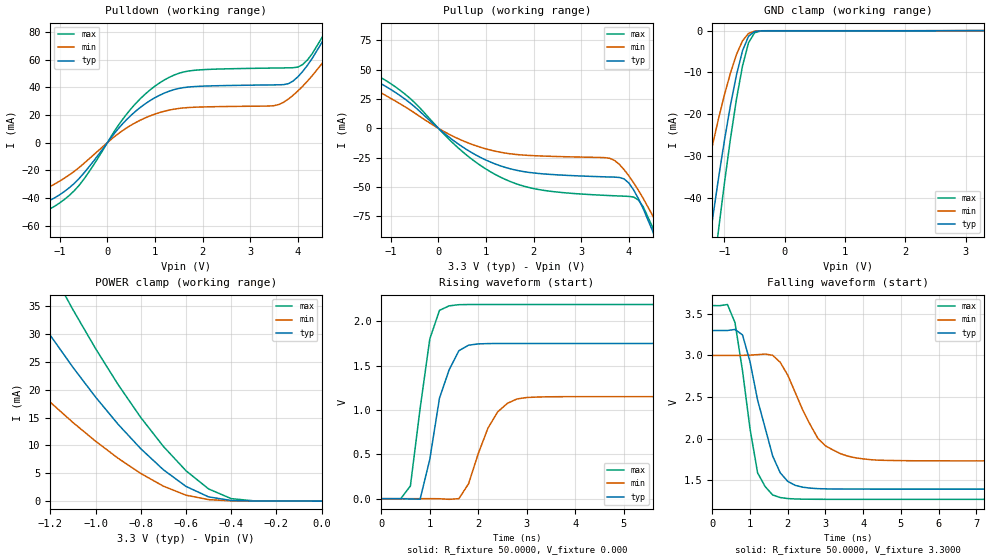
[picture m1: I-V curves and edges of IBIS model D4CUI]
| IBIS file t4i.ibs created by s2ibis2 version 1.1
| North Carolina State University Electronics Research Laboratory  1995
[IBIS ver]   2.1
[File name]   d4cui.ibs
[File Rev]   1.0
[Date]   Wednesday, March 29, 2000
[Source]   From silicon level SPICE at TOSHIBA.
[Notes]   This model does not include the values of Package Model
[Disclaimer]   None.
[Copyright]   Copyright(C) TOSHIBA Corp. 1996-2000. All Rights Reserved
|   Component TC260C
[Component]   TC260C
[Manufacturer]   TOSHIBA
[Package]
| variable   typ   min   max
R_pkg   1.00f   NA   NA
L_pkg   1.00fH   NA   NA
C_pkg   1.00fF   NA   NA
[Pin]  signal_name   model_name   R_pin   L_pin   C_pin
IO   IO   D4CUI
VDDS   VDDS   POWER
VSS   VSS   GND
| Models and submodels in the file (1): D4CUI (I/O)
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|   Model D4CUI
[Model]   D4CUI
Model_type   I/O
Polarity   Non-Inverting
Vinl   = 0.66V
Vinh   = 2.64V
C_comp   4.3pF   NA   NA
Vmeas = 1.65V
|Variable   typ   min   max
[Voltage range]  3.3   3.0   3.6
[Temperature Range]   25   100   0
[Pullup Reference]   3.3   3.0   3.6
[Pulldown Reference]   0.0   0.0   0.0
[POWER Clamp Reference]   3.3   3.0   3.6
[GND Clamp Reference]   0.0   0.0   0.0
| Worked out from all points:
|   slope of the pulldown table from 0 to 0.495 V, typ, clamps not added: 25.2 ohm
|   slope of the pullup table from 0 to 0.495 V, typ, clamps not added: 31.9 ohm
|   GND clamp passes 1 mA (typ) near -0.57 V on its own axis
|   POWER clamp passes 1 mA (typ) near -0.51 V on its own axis
|   rising waveform, R_fixture 50.0000, V_fixture 0.000: 20-80 % time 408ps typ, 500ps min, 320ps max; typ from 0 V to 1.75 V
|   falling waveform, R_fixture 50.0000, V_fixture 3.3000: 20-80 % time 615ps typ, 821ps min, 454ps max; typ from 3.3 V to 1.39 V
[Pulldown]
| voltage   I(typ)   I(min)   I(max)
-3.3V     -59mA      -58.31mA   -64.86mA
-1.9V     -51.23mA   -43.07mA   -57.58mA
-1V       -37.65mA   -27.81mA   -43.59mA
-500mV    -22.31mA   -15.25mA   -26.74mA
600mV     22.86mA    14.58mA    28.46mA
1.4V      38.26mA    24.15mA    48.77mA
3.6V      41.74mA    27.49mA    53.92mA
3.8V      42.56mA    31.44mA    54.02mA
4.1V      51.34mA    40.69mA    56.35mA
4.7V      84.91mA    66.18mA    89.44mA
5.1V      114.3mA    87.51mA    123mA
6.6V      274.3mA    211.8mA    309.5mA
[Pullup]
| voltage   I(typ)   I(min)   I(max)
-3.3V     71.91mA    86.68mA    73.87mA
-2.1V     55.22mA    51.34mA    59.93mA
-1.1V     35.6mA     27.85mA    40.67mA
-500mV    18.41mA    13.14mA    21.98mA
500mV     -15.68mA   -10.38mA   -19.73mA
1.5V      -34.43mA   -21.67mA   -45.26mA
3.7V      -41.64mA   -27.45mA   -57.55mA
4V        -46.74mA   -40.6mA    -58.07mA
4.2V      -60.02mA   -52.9mA    -61.17mA
4.5V      -87.85mA   -74.56mA   -84.58mA
4.7V      -109.3mA   -90.59mA   -107mA
6.6V      -337.2mA   -276.9mA   -360.7mA
[GND_clamp]
| voltage   I(typ)   I(min)   I(max)
-3.3V     -292.9mA   -217.9mA   -337.6mA
-1.5V     -78.02mA   -49.1mA    -99.03mA
-1.3V     -55.93mA   -34.39mA   -72.82mA
-1.2V     -45.48mA   -27.6mA    -60.2mA
-1.1V     -35.57mA   -21.25mA   -48.06mA
-900mV    -17.92mA   -10.17mA   -25.93mA
-800mV    -10.62mA   -5.728mA   -16.42mA
-700mV    -4.847mA   -2.443mA   -8.473mA
-600mV    -1.357mA   -679.2uA   -2.912mA
-500mV    -225.1uA   -138.4uA   -522.2uA
-400mV    -68.02uA   -43.8uA    -112uA
3.3V      153.9pA    14.42uA    -16.89uA
[POWER_clamp]
| voltage   I(typ)   I(min)   I(max)
-3.3V     189.3mA    136.1mA    229.5mA
-1.7V     62.67mA    39.14mA    83.1mA
-1.6V     55.64mA    34.47mA    74.42mA
-1.3V     35.82mA    21.61mA    49.54mA
-1.2V     29.75mA    17.75mA    41.78mA
-1.1V     24.02mA    14.12mA    34.37mA
-900mV    13.79mA    7.692mA    20.91mA
-800mV    9.41mA     4.966mA    15.02mA
-600mV    2.644mA    1.069mA    5.459mA
-500mV    763.5uA    269.3uA    2.188mA
-400mV    115.4uA    51.5uA     450.7uA
0V        153.9pA    711.8pA    166.4pA
[Ramp]
| variable   typ   min   max
dV/dt_r   1.0489/0.3314n   0.6897/0.4831n   1.3124/0.2690n
dV/dt_f   1.1453/0.5524n   0.7612/0.8651n   1.3990/0.4225n
R_load = 50.0000
[Rising Waveform]
R_fixture = 50.0000
V_fixture = 0.000
V_fixture_min = 0.000
V_fixture_max = 0.000
| time   V(typ)   V(min)   V(max)
0s        0V         0V         0V
600ps     -3.099mV   18.79uV    143.2mV
800ps     -5.757mV   124uV      1.014V
1ns       441.6mV    332.4uV    1.799V
1.2ns     1.132V     -520.1uV   2.121V
1.4ns     1.452V     -7.228mV   2.172V
1.8ns     1.729V     167.6mV    2.187V
2.2ns     1.747V     794.3mV    2.187V
2.8ns     1.748V     1.123V     2.187V
10ns      1.748V     1.149V     2.187V
[Falling Waveform]
R_fixture = 50.0000
V_fixture = 3.3000
V_fixture_min = 3.0000
V_fixture_max = 3.6000
| time   V(typ)   V(min)   V(max)
0s        3.3V       3V         3.6V
400ps     3.3V       3V         3.613V
600ps     3.312V     3V         3.396V
800ps     3.248V     3.001V     2.816V
1.2ns     2.463V     3.01V      1.588V
1.6ns     1.79V      3.002V     1.321V
2.2ns     1.437V     2.553V     1.273V
2.8ns     1.397V     2.002V     1.269V
3.4ns     1.392V     1.818V     1.268V
10ns      1.391V     1.731V     1.268V
